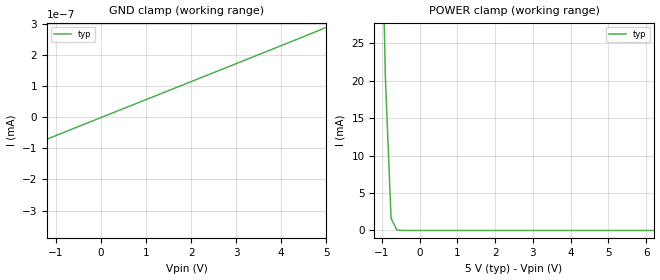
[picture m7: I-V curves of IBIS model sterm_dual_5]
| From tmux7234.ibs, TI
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| sterm_dual_5
[Model]   sterm_dual_5
Model_type   Terminator
|   typ   min   max
C_comp   6.362683e-12   NA   NA
[Voltage Range]   5   NA   NA
[Temperature Range]   27   NA   NA
[Power Clamp Reference]   5   NA   NA
[GND Clamp Reference]   0   NA   NA
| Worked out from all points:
|   GND clamp passes 1 mA (typ) near -5.70 V on its own axis
|   POWER clamp passes 1 mA (typ) near -0.70 V on its own axis
[GND Clamp]
|   Voltage   I(typ)   I(min)   I(max)
-10V      -2.114A    NA         NA
-5.152V   -611.1pA   NA         NA
-5V       -290.9pA   NA         NA
5V        288pA      NA         NA
[POWER Clamp]
|   Voltage   I(typ)   I(min)   I(max)
-5V       2.74A      NA         NA
-1.061V   58.05mA    NA         NA
-909.1mV  20.54mA    NA         NA
-757.6mV  1.616mA    NA         NA
-606.1mV  68.86uA    NA         NA
10V       -290.9pA   NA         NA
